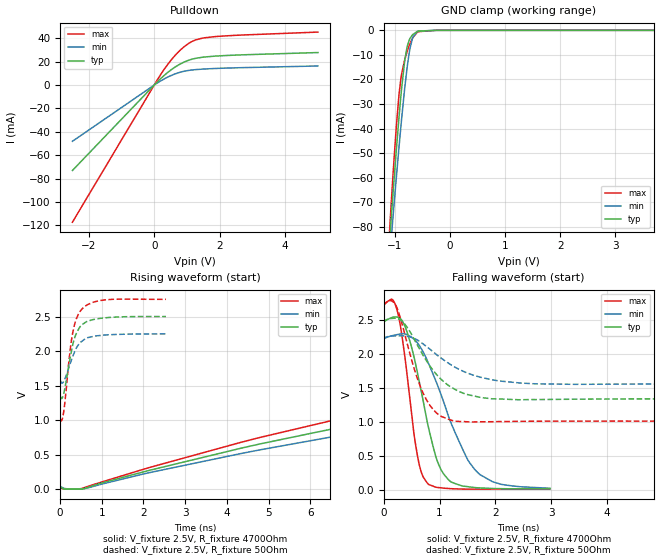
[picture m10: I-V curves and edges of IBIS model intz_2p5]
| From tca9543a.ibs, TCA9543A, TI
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|   intz_2p5 Model
[Model]   intz_2p5
Model_type   Open_drain
Polarity   Non-Inverting
Vmeas = 1.25
Vref = 2.5
Cref = 100pF
Rref = 4700
|   typ   min   max
|   (nom PVT)   (fast PVT)   (slow PVT)
C_comp   1.593e-12   1.501e-12   1.784e-12
| Where nom  PVT is Nominal Process, 2.5V, 27C
|   Fast PVT is Strong Process,  2.75V, -40C
|   Slow PVT is Weak Process,   2.25V, 85C
[Voltage Range]   2.5   2.25   2.75
|Junction Temperature
[Temperature Range]   27   85   -40
[Pullup Reference]   2.5   2.25   2.75
[Pulldown Reference]   0   0   0
[Power Clamp Reference]   2.5   2.25   2.75
[GND Clamp Reference]   0   0   0
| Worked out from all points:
|   slope of the pulldown table from 0 to 0.375 V, typ, clamps not added: 37.9 ohm
|   GND clamp passes 1 mA (typ) near -0.63 V on its own axis
|   falling waveform, V_fixture 2.5V, R_fixture 4700Ohm: 20-80 % time 397ps typ, 659ps min, 255ps max; typ from 2.5 V to 0.017 V
|   rising waveform, V_fixture 2.5V, R_fixture 4700Ohm: 20-80 % time 18.3ns typ, 19.2ns min, 17.5ns max; typ from 0.018 V to 2.5 V
|   falling waveform, V_fixture 2.5V, R_fixture 50Ohm: 20-80 % time 593ps typ, 802ps min, 404ps max; typ from 2.5 V to 1.34 V
|   rising waveform, V_fixture 2.5V, R_fixture 50Ohm: 20-80 % time 253ps typ, 289ps min, 223ps max; typ from 1.34 V to 2.5 V
[Pulldown]
|   Voltage   I(typ)   I(min)   I(max)
-2.5V     -73.08mA   -48.11mA   -117.3mA
162.5mV   4.588mA    2.944mA    7.499mA
357.3mV   9.497mA    6.021mA    15.57mA
599.2mV   14.65mA    9.106mA    24.13mA
951.3mV   20.11mA    12mA       33.56mA
1.268V    22.85mA    13.17mA    38.59mA
1.54V     23.96mA    13.71mA    40.38mA
1.849V    24.69mA    14.13mA    41.37mA
5V        27.76mA    16.28mA    45.26mA
[GND Clamp]
|   Voltage   I(typ)   I(min)   I(max)
-2.5V     -592.9mA   -541.2mA   -685mA
-1.155V   -105.5mA   -110.7mA   -104.8mA
-1.059V   -74.99mA   -83.61mA   -68.72mA
-1.03V    -66.14mA   -75.68mA   -58.45mA
-971mV    -48.78mA   -59.96mA   -39.17mA
-924.3mV  -35.89mA   -48mA      -26.67mA
-877.5mV  -24.2mA    -36.64mA   -18.15mA
-817mV    -12.13mA   -23.2mA    -11.81mA
-722.5mV  -3.275mA   -7.31mA    -5.359mA
-675mV    -1.731mA   -3.01mA    -3.09mA
-590mV    -465.8uA   -440.8uA   -787.4uA
5V        0A         0A         0A
[POWER Clamp]
|   Voltage   I(typ)   I(min)   I(max)
-2.5V     0A         0A         0A
-2.392V   0A         0A         0A
5V        0A         0A         0A
[Ramp]
R_load = 4700
|   typ   min   max
dV/dt_r   1.48923/1.82783e-08   1.33503/1.91855e-08   1.64273/1.74336e-08
dV/dt_f   1.48923/3.9643e-10   1.33503/6.59474e-10   1.64273/2.54522e-10
[Falling Waveform]
V_fixture = 2.5V
V_fixture_min = 2.25V
V_fixture_max = 2.75V
R_fixture = 4700Ohm
|   Time   V(typ)   V(min)   V(max)
0s        2.5V       2.25V      2.75V
150ps     2.535V     2.267V     2.802V
260ps     2.538V     2.287V     2.578V
410ps     2.342V     2.285V     1.755V
600ps     1.738V     2.168V     524.2mV
780ps     997.9mV    1.904V     101.8mV
940ps     472.3mV    1.591V     38.84mV
1.08ns    228.4mV    1.28V      24.86mV
1.68ns    30.98mV    258.2mV    10.64mV
2.98ns    17.14mV    23.63mV    12.5mV
[Rising Waveform]
V_fixture = 2.5V
V_fixture_min = 2.25V
V_fixture_max = 2.75V
R_fixture = 4700Ohm
|   Time   V(typ)   V(min)   V(max)
0s        17.95mV    24.95mV    12.12mV
540ps     0V         3.07mV     13.95mV
4.36ns    596.4mV    518.8mV    682.3mV
6.59ns    880.1mV    765.2mV    1.004V
11.63ns   1.386V     1.209V     1.571V
17.6ns    1.795V     1.575V     2.021V
25.03ns   2.112V     1.865V     2.362V
36.33ns   2.354V     2.096V     2.62V
46.28ns   2.446V     2.188V     2.712V
77.93ns   2.501V     2.25V      2.754V
[Falling Waveform]
V_fixture = 2.5V
V_fixture_min = 2.25V
V_fixture_max = 2.75V
R_fixture = 50Ohm
|   Time   V(typ)   V(min)   V(max)
0s        2.5V       2.25V      2.75V
230ps     2.522V     2.266V     2.694V
360ps     2.457V     2.266V     2.346V
590ps     2.15V      2.211V     1.669V
780ps     1.882V     2.1V       1.305V
970ps     1.676V     1.974V     1.114V
1.22ns    1.505V     1.832V     1.022V
1.74ns    1.359V     1.655V     1.002V
2.46ns    1.326V     1.571V     1.008V
6.84ns    1.34V      1.562V     1.011V
[Rising Waveform]
V_fixture = 2.5V
V_fixture_min = 2.25V
V_fixture_max = 2.75V
R_fixture = 50Ohm
|   Time   V(typ)   V(min)   V(max)
0s        1.339V     1.563V     1.011V
40ps      1.313V     1.535V     996.6mV
90ps      1.397V     1.567V     1.141V
230ps     1.87V      1.798V     1.962V
300ps     2.088V     1.917V     2.26V
390ps     2.258V     2.046V     2.47V
530ps     2.385V     2.146V     2.615V
780ps     2.456V     2.211V     2.706V
1.05ns    2.481V     2.232V     2.741V
2.54ns    2.501V     2.25V      2.75V
